| IBIS file stm32u073_083_ufbga81.ibs|
[IBIS ver] 4.2
[File name] stm32u073_083_ufbga81.ibs
[File Rev] 0.3
[Date] 20-02-2024
[Source] Data Created at STMicroelectronics
[Notes]  File originated from ELDO simulations.
[Disclaimer]  This information is for modeling purpose only and is
   not guaranteed. The information is subject to change without
   notice.
[Copyright] Copyright 2024 STMicroelectronics Inc.
|   Component stm32u073_083_ufbga81
[Component] stm32u073_083_ufbga81
[Manufacturer] STMicroelectronics
[Package]
| variable   typ   min   max
R_pkg  0  NA  NA
L_pkg  0  NA  NA
C_pkg  0  NA  NA
[Pin]   signal_name   model_name
A1  PB8  io8_ft_i2c
A2  PF3-BOOT0  io8_ft_v33
A3  PB4  io8_ft_i2c
A4  PB5  io8_ft
A5  PD4  io8_ft
A6  PD0  io8_ft
A7  PC12  io8_ft
A8  PC10  io8_ft
A9  PA15  io8_ft
B1  VBAT  power
B2  PB9  io8_ft_i2c
B3  PB7  io8_ft_i2c
B4  PB6  io8_ft_i2c
B5  PD6  io8_ft
B6  PD1  io8_ft
B7  PC11  io8_ft
B8  PA14  io8_ft
B9  PA13  io8_ft
C1  PC15-OSC32_OUT  io8_ft
C2  PC14-OSC32_IN  io8_ft_v33
C3  VDD12  nc
C4  PB3  io8_ft_i2c
C5  PD5  io8_ft
C6  PD2  io8_ft
C7  VDDUSB  power
C8  PA12  io8usb_ft_phy
C9  PA11  io8usb_ft_phy
D1  PF1-OSC_OUT  io8_ft
D2  PF0-OSC_IN  io8_ft
D3  VDD  power
D4  VSS  gnd
D5  PD3  io8_ft
D6  VSS  gnd
D7  PA9  io8_ft_i2c
D8  PA10  io8_ft_i2c
D9  PC9  io8_ft
E1  PC0  io8_ft_i2c
E2  PF2-NRST  ioreset_ft_v33
E3  PC13  io8_ft_v33
E4  PA1  io8_ft_v33
E5  PC8  io8_ft
E6  PC7  io8_ft
E7  PA8  io8_ft
E8  PC6  io8_ft
E9  PD13  io8_ft_i2c
F1  PC1  io8_ft_i2c
F2  PC2  io8_ft
F3  PA0  io8_ft_v33
F4  VSS  gnd
F5  PB0  io8_ft
F6  VSS  gnd
F7  PB15  io8_ft_v33
F8  PD11  io8_ft
F9  PD12  io8_ft_i2c
G1  PC3  io8_ft
G2  VSSA_VREFM  nc
G3  VDD  power
G4  PC5  io8_ft_v33
G5  PE7  io8_ft
G6  PE8  io8_ft
G7  VDD  power
G8  PD9  io8_ft
G9  PD10  io8_ft
H1  VREFP  nc
H2  PA2  io8_ft_v33
H3  PA5  io8_ft
H4  PA7  io8_ft_i2c
H5  PB1  io8_ft
H6  PE9  io8_ft
H7  PB11  io8_ft_i2c
H8  PB13  io8_ft_i2c
H9  PD8  io8_ft
J1  VDDA  nc
J2  PA3  io8_ft
J3  PA4  io8_ft
J4  PA6  io8_ft_i2c
J5  PC4  io8_ft
J6  PB2  io8_ft
J7  PB10  io8_ft_i2c
J8  PB12  io8_ft
J9  PB14  io8_ft_i2c
[Package Model]   489-ufbga-5x5-81-231214
[Pin Mapping]   pulldown_ref   pullup_ref   | Comment
A1  gndio  vddio
A2  gndio  vddio
A3  gndio  vddio
A4  gndio  vddio
A5  gndio  vddio
A6  gndio  vddio
A7  gndio  vddio
A8  gndio  vddio
A9  gndio  vddio
B1  nc  vsw
B2  gndio  vddio
B3  gndio  vddio
B4  gndio  vddio
B5  gndio  vddio
B6  gndio  vddio
B7  gndio  vddio
B8  gndio  vddio
B9  gndio  vddio
C1  gndio  vddio  | Depending on IO usage
| C1  gndio  vsw  | Depending on IO usage
C2  gndio  vddio  | Depending on IO usage
| C2  gndio  vsw  | Depending on IO usage
C3  nc  nc
C4  gndio  vddio
C5  gndio  vddio
C6  gndio  vddio
C7  nc  vddusb
C8  gndio  vddusb  | Depending on IO usage
| C8  gndio  vddio  | Depending on IO usage
C9  gndio  vddusb  | Depending on IO usage
| C9  gndio  vddio  | Depending on IO usage
D1  gndio  vddio
D2  gndio  vddio
D3  nc  vddio
D4  gndio  nc
D5  gndio  vddio
D6  gndio  nc
D7  gndio  vddio
D8  gndio  vddio
D9  gndio  vddio
E1  gndio  vddio
E2  gndio  vddio
E3  gndio  vddio  | Depending on IO usage
| E3  gndio  vsw  | Depending on IO usage
E4  gndio  vddio
E5  gndio  vddio
E6  gndio  vddio
E7  gndio  vddio
E8  gndio  vddio
E9  gndio  vddio
F1  gndio  vddio
F2  gndio  vddio
F3  gndio  vddio
F4  gndio  nc
F5  gndio  vddio
F6  gndio  nc
F7  gndio  vddio
F8  gndio  vddio
F9  gndio  vddio
G1  gndio  vddio
G2  nc  nc
G3  nc  vddio
G4  gndio  vddio
G5  gndio  vddio
G6  gndio  vddio
G7  nc  vddio
G8  gndio  vddio
G9  gndio  vddio
H1  nc  nc
H2  gndio  vddio
H3  gndio  vddio
H4  gndio  vddio
H5  gndio  vddio
H6  gndio  vddio
H7  gndio  vddio
H8  gndio  vddio
H9  gndio  vddio
J1  nc  nc
J2  gndio  vddio
J3  gndio  vddio
J4  gndio  vddio
J5  gndio  vddio
J6  gndio  vddio
J7  gndio  vddio
J8  gndio  vddio
J9  gndio  vddio
|[Diff Pin]   inv_pin   vdiff   tdelay_typ   tdelay_min   tdelay_max
|C8   C9   NA   NA   NA   NA
[Model Selector] io8_ft
io8_ft_ls_1v2   "GPIO - 5V tolerant - 1.2V range - Low speed"
io8_ft_ms_1v2   "GPIO - 5V tolerant - 1.2V range - Med speed"
io8_ft_fs_1v2   "GPIO - 5V tolerant - 1.2V range - Fast speed"
io8_ft_hs_1v2   "GPIO - 5V tolerant - 1.2V range - High speed"
io8_ft_ls_1v8   "GPIO - 5V tolerant - 1.8V range - Low speed"
io8_ft_ms_1v8   "GPIO - 5V tolerant - 1.8V range - Med speed"
io8_ft_fs_1v8   "GPIO - 5V tolerant - 1.8V range - Fast speed"
io8_ft_hs_1v8   "GPIO - 5V tolerant - 1.8V range - High speed"
io8_ft_ls_3v3   "GPIO - 5V tolerant - 3.3V range - Low speed"
io8_ft_ms_3v3   "GPIO - 5V tolerant - 3.3V range - Med speed"
io8_ft_fs_3v3   "GPIO - 5V tolerant - 3.3V range - Fast speed"
io8_ft_hs_3v3   "GPIO - 5V tolerant - 3.3V range - High speed"
[Model Selector] io8_ft_i2c
io8_ft_ls_1v2   "GPIO - 5V tolerant - 1.2V range - Low speed"
io8_ft_ms_1v2   "GPIO - 5V tolerant - 1.2V range - Med speed"
io8_ft_fs_1v2   "GPIO - 5V tolerant - 1.2V range - Fast speed"
io8_ft_hs_1v2   "GPIO - 5V tolerant - 1.2V range - High speed"
io8_ft_ls_1v8   "GPIO - 5V tolerant - 1.8V range - Low speed"
io8_ft_ms_1v8   "GPIO - 5V tolerant - 1.8V range - Med speed"
io8_ft_fs_1v8   "GPIO - 5V tolerant - 1.8V range - Fast speed"
io8_ft_hs_1v8   "GPIO - 5V tolerant - 1.8V range - High speed"
io8_ft_ls_3v3   "GPIO - 5V tolerant - 3.3V range - Low speed"
io8_ft_ms_3v3   "GPIO - 5V tolerant - 3.3V range - Med speed"
io8_ft_fs_3v3   "GPIO - 5V tolerant - 3.3V range - Fast speed"
io8_ft_hs_3v3   "GPIO - 5V tolerant - 3.3V range - High speed"
io8_ft_i2c_ls_1v2   "GPIO I2C open-drain - 5V tolerant - 1.2V range - Low speed"
io8_ft_i2c_ms_1v2   "GPIO I2C open-drain - 5V tolerant - 1.2V range - Med speed"
io8_ft_i2c_fs_1v2   "GPIO I2C open-drain - 5V tolerant - 1.2V range - Fast speed"
io8_ft_i2c_hs_1v2   "GPIO I2C open-drain - 5V tolerant - 1.2V range - High speed"
io8_ft_i2c_ls_1v8   "GPIO I2C open-drain - 5V tolerant - 1.8V range - Low speed"
io8_ft_i2c_ms_1v8   "GPIO I2C open-drain - 5V tolerant - 1.8V range - Med speed"
io8_ft_i2c_fs_1v8   "GPIO I2C open-drain - 5V tolerant - 1.8V range - Fast speed"
io8_ft_i2c_hs_1v8   "GPIO I2C open-drain - 5V tolerant - 1.8V range - High speed"
io8_ft_i2c_ls_3v3   "GPIO I2C open-drain - 5V tolerant - 3.3V range - Low speed"
io8_ft_i2c_ms_3v3   "GPIO I2C open-drain - 5V tolerant - 3.3V range - Med speed"
io8_ft_i2c_fs_3v3   "GPIO I2C open-drain - 5V tolerant - 3.3V range - Fast speed"
io8_ft_i2c_hs_3v3   "GPIO I2C open-drain - 5V tolerant - 3.3V range - High speed"
io8_ft_i2c_fmp_3v3   "GPIO I2C open-drain fm+ - 5V tolerant - 3.3V range"
[Model Selector] io8_ft_v33
io8_ft_v33_ls_1v2   "GPIO_V33 - 5V tolerant - 1.2V range - Low speed"
io8_ft_v33_ms_1v2   "GPIO_V33 - 5V tolerant - 1.2V range - Med speed"
io8_ft_v33_fs_1v2   "GPIO_V33 - 5V tolerant - 1.2V range - Fast speed"
io8_ft_v33_hs_1v2   "GPIO_V33 - 5V tolerant - 1.2V range - High speed"
io8_ft_v33_ls_1v8   "GPIO_V33 - 5V tolerant - 1.8V range - Low speed"
io8_ft_v33_ms_1v8   "GPIO_V33 - 5V tolerant - 1.8V range - Med speed"
io8_ft_v33_fs_1v8   "GPIO_V33 - 5V tolerant - 1.8V range - Fast speed"
io8_ft_v33_hs_1v8   "GPIO_V33 - 5V tolerant - 1.8V range - High speed"
io8_ft_v33_ls_3v3   "GPIO_V33 - 5V tolerant - 3.3V range - Low speed"
io8_ft_v33_ms_3v3   "GPIO_V33 - 5V tolerant - 3.3V range - Med speed"
io8_ft_v33_fs_3v3   "GPIO_V33 - 5V tolerant - 3.3V range - Fast speed"
io8_ft_v33_hs_3v3   "GPIO_V33 - 5V tolerant - 3.3V range - High speed"
[Model Selector] io8usb_ft_phy
io8_ft_ls_1v2   "GPIO - 5V tolerant - 1.2V range - Low speed"
io8_ft_ms_1v2   "GPIO - 5V tolerant - 1.2V range - Med speed"
io8_ft_fs_1v2   "GPIO - 5V tolerant - 1.2V range - Fast speed"
io8_ft_hs_1v2   "GPIO - 5V tolerant - 1.2V range - High speed"
io8_ft_ls_1v8   "GPIO - 5V tolerant - 1.8V range - Low speed"
io8_ft_ms_1v8   "GPIO - 5V tolerant - 1.8V range - Med speed"
io8_ft_fs_1v8   "GPIO - 5V tolerant - 1.8V range - Fast speed"
io8_ft_hs_1v8   "GPIO - 5V tolerant - 1.8V range - High speed"
io8_ft_ls_3v3   "GPIO - 5V tolerant - 3.3V range - Low speed"
io8_ft_ms_3v3   "GPIO - 5V tolerant - 3.3V range - Med speed"
io8_ft_fs_3v3   "GPIO - 5V tolerant - 3.3V range - Fast speed"
io8_ft_hs_3v3   "GPIO - 5V tolerant - 3.3V range - High speed"
io8usb_ft_phy_hs_3v3   "USB full speed"
io8usb_ft_phy_ls_3v3   "USB low speed"
[Model Selector] ioreset_ft_v33
ioreset_ft_v33_1v2   "Reset PAD. 5V tolerant. 1.2V range"
ioreset_ft_v33_1v8   "Reset PAD. 5V tolerant. 1.8V range"
ioreset_ft_v33_3v3   "Reset PAD. 5V tolerant. 3.3V range"
[Define Package Model]  489-ufbga-5x5-81-231214
[Manufacturer]  unknown
[OEM]  unknown
[Description]  unknown
[Number Of Pins]  76
[Pin Numbers]
| Pin Name Terminal   Net Name   Starting Node   Ending Node
F3 | PA0
E4 | PA1
H2 | PA2
J2 | PA3
J3 | PA4
H3 | PA5
J4 | PA6
H4 | PA7
E7 | PA8
D7 | PA9
D8 | PA10
C9 | PA11
C8 | PA12
B9 | PA13
B8 | PA14
A9 | PA15
F5 | PB0
H5 | PB1
J6 | PB2
C4 | PB3
A3 | PB4
A4 | PB5
B4 | PB6
B3 | PB7
A1 | PB8
B2 | PB9
J7 | PB10
H7 | PB11
J8 | PB12
H8 | PB13
J9 | PB14
F7 | PB15
E1 | PC0
F1 | PC1
F2 | PC2
G1 | PC3
J5 | PC4
G4 | PC5
E8 | PC6
E6 | PC7
E5 | PC8
D9 | PC9
A8 | PC10
B7 | PC11
A7 | PC12
E3 | PC13
C2 | PC14-OSC32_IN
C1 | PC15-OSC32_OUT
A6 | PD0
B6 | PD1
C6 | PD2
D5 | PD3
A5 | PD4
C5 | PD5
B5 | PD6
H9 | PD8
G8 | PD9
G9 | PD10
F8 | PD11
F9 | PD12
E9 | PD13
G5 | PE7
G6 | PE8
H6 | PE9
D2 | PF0-OSC_IN
D1 | PF1-OSC_OUT
E2 | PF2-NRST
A2 | PF3-BOOT0
B1 | VBAT
C3 | VDD12
D3 | VDD
J1 | VDDA
C7 | VDDUSB
H1 | VREFP
D4 | VSS
G2 | VSSA_VREFM
|[Merged Pins]  D3
|G3  |  VDD
|G7  |  VDD
|[Merged Pins]  D4
|D6  |  VSS
|F4  |  VSS
|F6  |  VSS
[Model Data]
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[End Model Data]
[End Package Model]
|End [Component]
| Models and submodels in the file (42): io8_ft_fs_1v2 (I/O), io8_ft_fs_1v8 (I/O), io8_ft_fs_3v3 (I/O), io8_ft_hs_1v2 (I/O), io8_ft_hs_1v8 (I/O), io8_ft_hs_3v3 (I/O), io8_ft_i2c_fmp_3v3 (I/O_open_drain), io8_ft_i2c_fs_1v2 (I/O_open_drain), io8_ft_i2c_fs_1v8 (I/O_open_drain), io8_ft_i2c_fs_3v3 (I/O_open_drain), io8_ft_i2c_hs_1v2 (I/O_open_drain), io8_ft_i2c_hs_1v8 (I/O_open_drain), io8_ft_i2c_hs_3v3 (I/O_open_drain), io8_ft_i2c_ls_1v2 (I/O_open_drain), io8_ft_i2c_ls_1v8 (I/O_open_drain), io8_ft_i2c_ls_3v3 (I/O_open_drain), io8_ft_i2c_ms_1v2 (I/O_open_drain), io8_ft_i2c_ms_1v8 (I/O_open_drain), io8_ft_i2c_ms_3v3 (I/O_open_drain), io8_ft_ls_1v2 (I/O), io8_ft_ls_1v8 (I/O), io8_ft_ls_3v3 (I/O), io8_ft_ms_1v2 (I/O), io8_ft_ms_1v8 (I/O), io8_ft_ms_3v3 (I/O), io8_ft_v33_fs_1v2 (I/O), io8_ft_v33_fs_1v8 (I/O), io8_ft_v33_fs_3v3 (I/O), io8_ft_v33_hs_1v2 (I/O), io8_ft_v33_hs_1v8 (I/O), io8_ft_v33_hs_3v3 (I/O), io8_ft_v33_ls_1v2 (I/O), io8_ft_v33_ls_1v8 (I/O), io8_ft_v33_ls_3v3 (I/O), io8_ft_v33_ms_1v2 (I/O), io8_ft_v33_ms_1v8 (I/O), io8_ft_v33_ms_3v3 (I/O), io8usb_ft_phy_hs_3v3 (I/O), io8usb_ft_phy_ls_3v3 (I/O), ioreset_ft_v33_1v2 (I/O_open_drain), ioreset_ft_v33_1v8 (I/O_open_drain), ioreset_ft_v33_3v3 (I/O_open_drain)
